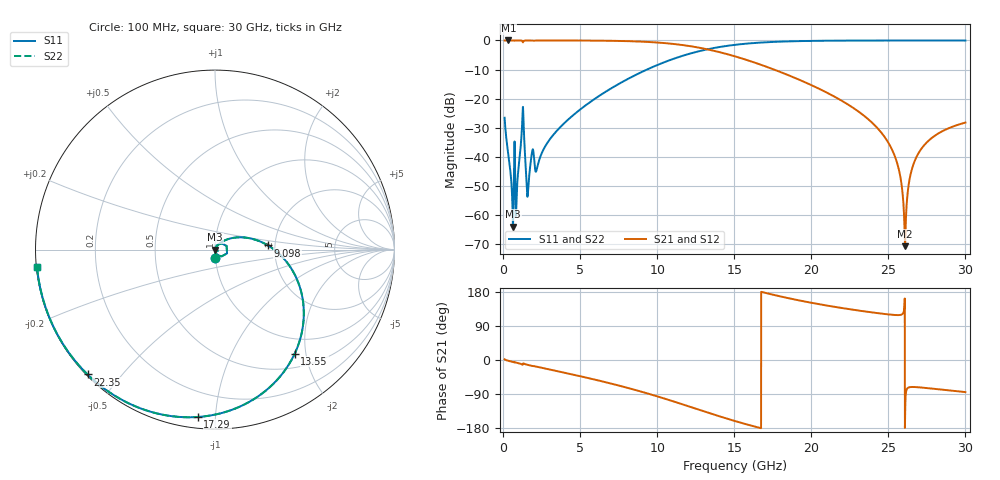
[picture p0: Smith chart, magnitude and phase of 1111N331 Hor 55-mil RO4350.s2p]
# GHz S MA R 50
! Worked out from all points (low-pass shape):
!   3201 points, 100 MHz to 30 GHz, reference 50 ohm
!   highest |S21| = 0.00 dB at 342.9 MHz (marker M1); lowest = -70.6 dB at 26.08 GHz (marker M2)
!   |S21| within 3 dB of the highest: start of sweep to 13.22 GHz
!   lowest |S11| = -63.9 dB at 641.9 MHz (marker M3), VSWR 1.00, Z = 50.1 - j0.0158 ohm
!   |S11| at or under -10 dB: start of sweep to 9.331 GHz
!   |S22| runs from -63.9 to 0.0 dB; largest |S21 - S12| = 0
!   S11 on the Smith chart (normalised r, x): 100 MHz: 1.00, -0.09; 9.098 GHz: 1.83, +0.09; 13.55 GHz: 0.73, -1.80; 17.29 GHz: 0.06, -0.90; 22.35 GHz: 0.00, -0.41; 30 GHz: 0.00, -0.05
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0.1  0.04714 -87.8  0.9986 1.9  0.9986 1.9  0.04714 -87.8
0.3429375  0.01096 -90.1  0.9995 -2.1  0.9995 -2.1  0.01096 -90.1
0.6419375  0.0006405 -14.2  0.9993 -5.1  0.9993 -5.1  0.0006405 -14.2
0.9409375  0.004232 70.7  0.999 -7.8  0.999 -7.8  0.004232 70.7
1.249281  0.04436 47.9  0.977 -12.2  0.977 -12.2  0.04436 47.9
1.623031  0.002625 27.4  0.9978 -13.1  0.9978 -13.1  0.002625 27.4
1.884656  0.01238 38.7  0.9925 -15.6  0.9925 -15.6  0.01238 38.7
2.193  0.006231 44.2  0.9968 -17.8  0.9968 -17.8  0.006231 44.2
5.089563  0.06804 45.2  0.9957 -43.6  0.9957 -43.6  0.06804 45.2
9.098031  0.2961 4.5  0.9517 -85.0  0.9517 -85.0  0.2961 4.5
10.06978  0.3844 -7.1  0.9192 -96.7  0.9192 -96.7  0.3844 -7.1
13.54566  0.7301 -52.5  0.6773 -142.2  0.6773 -142.2  0.7301 -52.5
15.05  0.8413 -71.4  0.5334 -161.1  0.5334 -161.1  0.8413 -71.4
17.2925  0.9375 -95.9  0.3381 174.4  0.3381 174.4  0.9375 -95.9
20.03956  0.9826 -119.6  0.1695 150.7  0.1695 150.7  0.9826 -119.6
22.34747  0.994 -135.6  0.08062 134.9  0.08062 134.9  0.994 -135.6
25.01978  0.9972 -151.0  0.01724 120.2  0.01724 120.2  0.9972 -151.0
25.67384  0.9973 -154.4  0.006221 118.5  0.006221 118.5  0.9973 -154.4
26.08497  0.9973 -156.5  0.0002951 -154.2  0.0002951 -154.2  0.9973 -156.5
26.47741  0.9973 -158.5  0.005497 -71.3  0.005497 -71.3  0.9973 -158.5
27.06606  0.9972 -161.3  0.01293 -72.4  0.01293 -72.4  0.9972 -161.3
30  0.9965 -174.5  0.03895 -84.7  0.03895 -84.7  0.9965 -174.5
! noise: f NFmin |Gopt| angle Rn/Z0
0.1  0.0006745  0.7374  0.9295  0.0005138
3.417  0.00936  0.4656  26.56  0.00282
6.743  0.01566  0.419  48.47  0.003785
10.06  0.02425  0.4644  66.42  0.00565
13.39  0.03833  0.5704  83.61  0.009501
16.7  0.06659  0.7143  102.7  0.01873
20.03  0.1389  0.8515  123  0.04636
23.35  0.4307  0.9492  142.3  0.2005
26.67  2.815  0.9916  159.4  2.618
30  0.6197  0.9616  174.5  0.009964
